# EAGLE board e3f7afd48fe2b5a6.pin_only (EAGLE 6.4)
REV: B

Size 17.78 x 28.57 mm. Coordinates in mm from the lower left corner, seen from the top.
Outline: 6.35,28.57 11.43,28.57
Outline: 0,0 0,26.04 arc-90 1.91,27.94 15.88,27.94 arc-90 17.78,26.04 17.78,0 0,0
Copper layers (1*16): Top 0.035mm / dielectric 1.5mm / Bottom 0.035mm
Design rules "adafruit *": minimum track width 8mil, minimum drill 15.5mil, track to track 8mil, track to pad 8mil, pad to pad 8mil, via to via 8mil, smd to smd 8mil, copper to edge 10mil, drill to drill 8mil, minimum pad ring 10mil, minimum via ring 8mil, stop-mask expansion 2mil, vias tented up to drill 20mil, thermal gap 10mil

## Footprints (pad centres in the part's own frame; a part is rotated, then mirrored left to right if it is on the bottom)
0805-NO = smd 1.3 x 1.5: 1 -0.95,0; 2 0.95,0
CHIPLED_0805_NOOUTLINE = smd 1.2 x 1.2: A 0,-1.05; C 0,1.05
FIDUCIAL_1MM = smd 1 x 1: 1 0,0
1X06_ROUND_76 = drill 1 pad 1.93: 1 -6.35,0; 2 -3.81,0; 3 -1.27,0; 4 1.27,0; 5 3.81,0; 6 6.35,0
1X08_ROUND_70 = drill 1 pad 1.778: 1 -8.89,0; 2 -6.35,0; 3 -3.81,0; 4 -1.27,0; 5 1.27,0; 6 3.81,0; 7 6.35,0; 8 8.89,0
QFN24_4MM_SMSC = smd 0.8 x 0.28: 1 -2,1.25; 2 -2,0.75; 3 -2,0.25; 4 -2,-0.25; 5 -2,-0.75; 6 -2,-1.25; 13 2,-1.25; 14 2,-0.75; 15 2,-0.25; 16 2,0.25; 17 2,0.75; 18 2,1.25 | smd 0.28 x 0.8: 7 -1.25,-2; 8 -0.75,-2; 9 -0.25,-2; 10 0.25,-2; 11 0.75,-2; 12 1.25,-2; 19 1.25,2; 20 0.75,2; 21 0.25,2; 22 -0.25,2; 23 -0.75,2; 24 -1.25,2 | smd 2.5 x 2.5: THERM 0,0
MOUNTINGHOLE_2.0_PLATED = drill 2.2 pad 3: P$1 0,0
4UCONN_20329_V2 = smd 1 x 2: BASE@1 -0.75,-2; BASE@2 0.75,-2 | smd 0.4 x 1.35: D+ 0,0.775; D- -0.65,0.775; GND 1.3,0.775; ID 0.65,0.775; VBUS -1.3,0.775 | drill 0.8 pad 1.2 offset: SPRT@1 -3.3,0.9; SPRT@2 3.3,0.9 | drill 0.9 pad 2.5 square: SPRT@3 -3.6,-1.9; SPRT@4 3.6,-1.9 | hole 0.7: -1.95,0; 1.95,0

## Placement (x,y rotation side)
C1  10uF  [0805-NO]  11.18,19.05 180 top
C2  10uF  [0805-NO]  11.18,21.21 0 top
C3  10uF  [0805-NO]  5.71,17.4 270 top
C4  0.1uF  [0805-NO]  5.71,20.83 270 top
D1  RED  [CHIPLED_0805_NOOUTLINE]  9.91,6.6 0 top
D2  GREEN  [CHIPLED_0805_NOOUTLINE]  8,6.6 0 top
FID1  FIDUCIAL""  [FIDUCIAL_1MM]  0.89,3.94 0 top
FID2  FIDUCIAL""  [FIDUCIAL_1MM]  7.49,20.83 0 top
JP1  FTDI  [1X06_ROUND_76]  8.89,2.54 0 top
JP2  Modem  [1X08_ROUND_70]  15.24,13.97 90 top
JP4  Control  [1X08_ROUND_70]  2.54,13.97 270 top
R1  1K  [0805-NO]  11.68,6.6 90 top
R2  1K  [0805-NO]  6.1,6.6 90 top
U1  CP2104  [QFN24_4MM_SMSC]  8.89,13.72 270 top
U$8  [ADAFRUIT_2.5MM]  7.24,16.76 0 top
U$17  [PCBFEAT-REV-040]  8.89,25.78 0 bottom
U$18  MOUNTINGHOLE2.0  [MOUNTINGHOLE_2.0_PLATED]  15.75,25.91 0 top
U$19  MOUNTINGHOLE2.0  [MOUNTINGHOLE_2.0_PLATED]  2.03,25.91 0 top
U$22  [ADAFRUIT_5MM]  11.18,7.24 0 bottom
X1  20329  [4UCONN_20329_V2]  8.89,24.38 180 top

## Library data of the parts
C1-C4 D1 D2 JP1 JP2 JP4 R1 R2 U1 U$8 U$17 U$22 X1 = microbuilder
FID1 FID2 U$18 U$19 = microbuilder; BOM: EXCLUDE

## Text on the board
tPlace: 5V | RI | 3Vo | DCD | GND | DTR | RST | DSR | IO3 | TXD | CP2104 | IO2 | RXD | R | T | RTS | #SU | SU | CTS | 5V | RXD | GND | CTS | TXD | RTS
bPlace: CP2104 / USB Serial | 3.3V Logic / 5V Tolerant / 300-2Mbps | FTDI compat / header pins

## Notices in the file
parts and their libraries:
microbuilder: This work is placed in the public domain, and may be freely used for commercial and non-commercial work with the following conditions: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
